| TEXAS INSTRUMENTS INCORPORATED
| Standard Linear and Logic Group
| IBIS Model of SN74CB3T16210
| 20-BIT FET BUS SWITCH 2.5-V/3.3-V LOW-VOLTAGE BUS SWITCH
| WITH 5-V TOLERANT/LEVEL SHIFTER
| This file contains package information for the following:
|  TSSOP 48-pin (DGG) package as [Component] CB3T16210_DGG
|  TVSOP 48-pin (DGV) package as [Component] CB3T16210_DGV
| This device can be powered at the following Vccs:
|  3.3 volt Vcc
|  2.5 volt Vcc
| This file provides unique models under the [Model Selector] for each Vcc.
| For operation at a specific Vcc, select the appropriate model after each
| [Model Selector] keyword.
[IBIS Ver]   3.2
[Comment char]  |_char
[File Name]   sn74cb3t16210.ibs
[File Rev]   1.1 | c_die
[Date]   April 30, 2004
[Source]   Data created from TI-SPICE simulations at TI-SLL.
[Notes]   The following is an IBIS list for the CB3T16210.
   Please contact sllibis@ti.com with questions and
   comments concerning SLL IBIS models.
   - FILE REV HISTORY
   - 1.1 Release IBIS file on 06/01/04
   - Non-monotonic data due to FET characteristics.
   - Power clamp data deleted as there is no power-clamp diode.
[Disclaimer] Property of Texas Instruments Incorporated.  Unauthorized
   reproduction and/or distribution is strictly prohibited.
   This product is protected under copyright law.
   Created  2003, (C) Copyright  2003, Texas Instruments
   Incorporated, All Rights Reserved
   UNLESS THERE IS A SIGNED, WRITTEN AGREEMENT TO THE
   CONTRARY, TEXAS INSTRUMENTS (TI) IS PROVIDING THE IBIS
   MODELS  AND WITHOUT ANY WARRANTY, EXPRESSED OR
   IMPLIED.  TI assumes no liability for:
   1) the accuracy of the IBIS models provided to your
   company;
   2) the proper functioning of these IBIS Models in your
   design or for any resulting applications; or
   3) infringement of patents, copyrights or intellectual
   property rights resulting from your use of these IBIS
   models.
   TI provides IBIS Models as a service to our customers.
   You and your company shall not distribute, sell or give
   these models to anyone else without prior written
   permission from TI.
   TI reserves the right to make changes to our products or
   to discontinue any semiconductor product or service
   without notice, and advises our customers to obtain the
   latest version of relevant information to verify, before
   placing orders, that the information being relied on is
   current.
   Please be aware that your receipt and use of the IBIS
   information provided shall serve as acceptance of these
   terms and conditions.  If you do not accept these terms,
   you should return or destroy the IBIS models and any
   other accompanying information immediately.
| Component CB3T16210_DGG 48-pin TSSOP
[Component]   CB3T16210_DGG
[Manufacturer]   Texas Instruments, Inc.
[Package]
|   typ   min   max
R_pkg   4.400e-02   3.800e-02   5.100e-02
L_pkg   3.019e-09   2.486e-09   4.099e-09
C_pkg   5.070e-13   3.340e-13   8.090e-13
[Pin]   signal_name   model_name   R_pin   L_pin   C_pin
1   NC   NC   4.100e-02   4.017e-09   7.590e-13
2   1A1   CB3T16210_IO   4.200e-02   3.737e-09   7.920e-13
3   1A2   CB3T16210_IO   4.200e-02   3.480e-09   6.610e-13
4   1A3   CB3T16210_IO   3.800e-02   3.131e-09   5.750e-13
5   1A4   CB3T16210_IO   4.700e-02   3.122e-09   5.660e-13
6   1A5   CB3T16210_IO   4.300e-02   2.948e-09   5.040e-13
7   1A6   CB3T16210_IO   4.500e-02   2.845e-09   3.970e-13
8   GND   GND   4.900e-02   2.835e-09   3.940e-13
9   1A7   CB3T16210_IO   4.800e-02   2.715e-09   3.780e-13
10   1A8   CB3T16210_IO   5.000e-02   2.664e-09   3.630e-13
11   1A9   CB3T16210_IO   5.000e-02   2.585e-09   3.480e-13
12   1A10   CB3T16210_IO   4.900e-02   2.550e-09   3.370e-13
13   2A1   CB3T16210_IO   4.900e-02   2.541e-09   3.360e-13
14   2A2   CB3T16210_IO   5.000e-02   2.574e-09   3.480e-13
15   VCC   POWER   4.900e-02   2.618e-09   3.590e-13
16   2A3   CB3T16210_IO   4.600e-02   2.671e-09   3.750e-13
17   GND   GND   4.500e-02   2.754e-09   3.890e-13
18   2A4   CB3T16210_IO   4.400e-02   2.823e-09   4.500e-13
19   2A5   CB3T16210_IO   4.200e-02   2.968e-09   5.030e-13
20   2A6   CB3T16210_IO   5.100e-02   3.108e-09   5.350e-13
21   2A7   CB3T16210_IO   4.200e-02   3.175e-09   5.870e-13
22   2A8   CB3T16210_IO   4.100e-02   3.449e-09   6.780e-13
23   2A9   CB3T16210_IO   4.400e-02   3.766e-09   8.040e-13
24   2A10   CB3T16210_IO   4.300e-02   4.065e-09   7.610e-13
25   2B10   CB3T16210_IO   4.100e-02   3.994e-09   7.570e-13
26   2B9   CB3T16210_IO   3.900e-02   3.649e-09   7.890e-13
27   2B8   CB3T16210_IO   3.800e-02   3.362e-09   6.600e-13
28   2B7   CB3T16210_IO   3.800e-02   3.082e-09   5.740e-13
29   2B6   CB3T16210_IO   4.400e-02   2.990e-09   5.220e-13
30   2B5   CB3T16210_IO   4.100e-02   2.917e-09   4.950e-13
31   2B4   CB3T16210_IO   4.300e-02   2.820e-09   4.480e-13
32   GND   GND   4.300e-02   2.699e-09   3.850e-13
33   2B3   CB3T16210_IO   4.500e-02   2.628e-09   3.720e-13
34   2B2   CB3T16210_IO   4.600e-02   2.556e-09   3.560e-13
35   2B1   CB3T16210_IO   4.600e-02   2.495e-09   3.440e-13
36   1B10   CB3T16210_IO   4.700e-02   2.487e-09   3.340e-13
37   1B9   CB3T16210_IO   4.700e-02   2.490e-09   3.350e-13
38   1B8   CB3T16210_IO   4.600e-02   2.486e-09   3.430e-13
39   1B7   CB3T16210_IO   4.500e-02   2.566e-09   3.560e-13
40   1B6   CB3T16210_IO   4.400e-02   2.639e-09   3.740e-13
41   GND   GND   4.300e-02   2.701e-09   3.860e-13
42   1B5   CB3T16210_IO   4.300e-02   2.817e-09   4.500e-13
43   1B4   CB3T16210_IO   4.100e-02   2.935e-09   5.010e-13
44   1B3   CB3T16210_IO   4.700e-02   3.035e-09   5.290e-13
45   1B2   CB3T16210_IO   4.300e-02   3.171e-09   5.890e-13
46   1B1   CB3T16210_IO   4.000e-02   3.415e-09   6.820e-13
47   NOE2   CB3T16210_IN   4.300e-02   3.741e-09   8.090e-13
48   NOE1   CB3T16210_IN   4.400e-02   4.099e-09   7.640e-13
| Component CB3T16210_DGV 48-pin TVSOP
[Component]   CB3T16210_DGV
[Manufacturer]   Texas Instruments, Inc.
[Package]
|   typ   min   max
R_pkg   7.000e-02   4.900e-02   8.500e-02
L_pkg   3.013e-09   2.743e-09   3.408e-09
C_pkg   3.710e-13   2.940e-13   5.110e-13
[Pin]   signal_name   model_name   R_pin   L_pin   C_pin
1   NC   NC   4.900e-02   3.393e-09   4.970e-13
2   1A1   CB3T16210_IO   6.000e-02   3.250e-09   5.020e-13
3   1A2   CB3T16210_IO   7.700e-02   3.310e-09   4.510e-13
4   1A3   CB3T16210_IO   8.500e-02   3.299e-09   4.040e-13
5   1A4   CB3T16210_IO   8.300e-02   3.136e-09   3.600e-13
6   1A5   CB3T16210_IO   7.700e-02   3.019e-09   3.630e-13
7   1A6   CB3T16210_IO   6.500e-02   2.882e-09   3.490e-13
8   GND   GND   6.600e-02   2.829e-09   3.140e-13
9   1A7   CB3T16210_IO   6.700e-02   2.796e-09   3.140e-13
10   1A8   CB3T16210_IO   6.900e-02   2.754e-09   3.080e-13
11   1A9   CB3T16210_IO   7.000e-02   2.753e-09   3.010e-13
12   1A10   CB3T16210_IO   7.100e-02   2.745e-09   2.940e-13
13   2A1   CB3T16210_IO   7.000e-02   2.744e-09   2.940e-13
14   2A2   CB3T16210_IO   7.000e-02   2.754e-09   3.010e-13
15   VCC   POWER   6.900e-02   2.754e-09   3.080e-13
16   2A3   CB3T16210_IO   6.700e-02   2.796e-09   3.140e-13
17   GND   GND   6.600e-02   2.829e-09   3.140e-13
18   2A4   CB3T16210_IO   6.500e-02   2.883e-09   3.500e-13
19   2A5   CB3T16210_IO   7.500e-02   3.014e-09   3.630e-13
20   2A6   CB3T16210_IO   8.000e-02   3.128e-09   3.580e-13
21   2A7   CB3T16210_IO   8.400e-02   3.295e-09   4.030e-13
22   2A8   CB3T16210_IO   7.800e-02   3.311e-09   4.520e-13
23   2A9   CB3T16210_IO   6.200e-02   3.259e-09   5.010e-13
24   2A10   CB3T16210_IO   5.200e-02   3.404e-09   4.960e-13
25   2B10   CB3T16210_IO   5.300e-02   3.397e-09   5.050e-13
26   2B9   CB3T16210_IO   6.200e-02   3.249e-09   5.110e-13
27   2B8   CB3T16210_IO   7.700e-02   3.308e-09   4.530e-13
28   2B7   CB3T16210_IO   8.200e-02   3.289e-09   4.030e-13
29   2B6   CB3T16210_IO   7.800e-02   3.121e-09   3.590e-13
30   2B5   CB3T16210_IO   7.400e-02   3.010e-09   3.630e-13
31   2B4   CB3T16210_IO   6.500e-02   2.883e-09   3.490e-13
32   GND   GND   6.700e-02   2.829e-09   3.140e-13
33   2B3   CB3T16210_IO   6.700e-02   2.795e-09   3.140e-13
34   2B2   CB3T16210_IO   6.900e-02   2.753e-09   3.070e-13
35   2B1   CB3T16210_IO   7.000e-02   2.753e-09   3.010e-13
36   1B10   CB3T16210_IO   7.000e-02   2.743e-09   2.940e-13
37   1B9   CB3T16210_IO   7.000e-02   2.743e-09   2.940e-13
38   1B8   CB3T16210_IO   7.000e-02   2.753e-09   3.010e-13
39   1B7   CB3T16210_IO   6.900e-02   2.754e-09   3.070e-13
40   1B6   CB3T16210_IO   6.800e-02   2.797e-09   3.140e-13
41   GND   GND   6.700e-02   2.830e-09   3.140e-13
42   1B5   CB3T16210_IO   6.400e-02   2.880e-09   3.490e-13
43   1B4   CB3T16210_IO   7.200e-02   3.004e-09   3.620e-13
44   1B3   CB3T16210_IO   7.800e-02   3.121e-09   3.590e-13
45   1B2   CB3T16210_IO   8.400e-02   3.296e-09   4.030e-13
46   1B1   CB3T16210_IO   7.700e-02   3.308e-09   4.510e-13
47   NOE2   CB3T16210_IN   6.200e-02   3.258e-09   4.990e-13
48   NOE1   CB3T16210_IN   5.300e-02   3.408e-09   4.940e-13
[Series Switch Groups]
| Function Group States
On  1 /   | 1A1-1A10->1B1-1B10 NOE1 LOW
On  2 /   | 2A1-2A10->2B1-2B10 NOE2 LOW
On  1 2 /   | Enable Both
Off 1 /   | 1A1-1A10->1B1-1B10 NOE1 HIGH
Off 2 /   | 2A1-2A10->2B1-2B10 NOE2 HIGH
Off 1 2 /   | Disable Both
[Series Pin Mapping]   pin_2   model_name   function_table_group
2   46   CB3T16210_IO_33_S   1
| 2   46   CB3T16210_IO_25_S   1
3   45   CB3T16210_IO_33_S   1
| 3   45   CB3T16210_IO_25_S   1
4   44   CB3T16210_IO_33_S   1
| 4   44   CB3T16210_IO_25_S   1
5   43   CB3T16210_IO_33_S   1
| 5   43   CB3T16210_IO_25_S   1
6   42   CB3T16210_IO_33_S   1
| 6   42   CB3T16210_IO_25_S   1
7   40   CB3T16210_IO_33_S   1
| 7   40   CB3T16210_IO_25_S   1
9   39   CB3T16210_IO_33_S   1
| 9   39   CB3T16210_IO_25_S   1
10   38   CB3T16210_IO_33_S   1
| 10   38   CB3T16210_IO_25_S   1
11   37   CB3T16210_IO_33_S   1
| 11   37   CB3T16210_IO_25_S   1
12   36   CB3T16210_IO_33_S   1
| 12   36   CB3T16210_IO_25_S   1
13   35   CB3T16210_IO_33_S   2
| 13   35   CB3T16210_IO_25_S   2
14   34   CB3T16210_IO_33_S   2
| 14   34   CB3T16210_IO_25_S   2
16   33   CB3T16210_IO_33_S   2
| 16   33   CB3T16210_IO_25_S   2
18   31   CB3T16210_IO_33_S   2
| 18   31   CB3T16210_IO_25_S   2
19   30   CB3T16210_IO_33_S   2
| 19   30   CB3T16210_IO_25_S   2
20   29   CB3T16210_IO_33_S   2
| 20   29   CB3T16210_IO_25_S   2
21   28   CB3T16210_IO_33_S   2
| 21   28   CB3T16210_IO_25_S   2
22   27   CB3T16210_IO_33_S   2
| 22   27   CB3T16210_IO_25_S   2
23   26   CB3T16210_IO_33_S   2
| 23   26   CB3T16210_IO_25_S   2
24   25   CB3T16210_IO_33_S   2
| 24   25   CB3T16210_IO_25_S   2
| Model CB3T16210_IN
[Model Selector]   CB3T16210_IN
CB3T16210_IN_33   3.3 volt Vcc
CB3T16210_IN_25   2.5 volt Vcc
| Model CB3T16210_IO
[Model Selector]   CB3T16210_IO
CB3T16210_IO_33   3.3 volt Vcc
CB3T16210_IO_25   2.5 volt Vcc
| Model CB3T16210_IO_S
[Model Selector]   CB3T16210_IO_S
CB3T16210_IO_33_S   3.3 volt Vcc_S
CB3T16210_IO_25_S   2.5 volt Vcc_S
[Model]   CB3T16210_IO_33_S
Model_type  Series_switch
| variable   typ   min   max
C_comp   0   0   0
[Temperature Range]   40   100   -40
| Ambient temperature   25   85   -40
[Voltage range]   3.3   3   3.6
[On]
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[Off]
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[Model]   CB3T16210_IO_25_S
Model_type  Series_switch
| variable   typ   min   max
C_comp   0   0   0
[Temperature Range]   40   100   -40
| Ambient temperature   25   85   -40
[Voltage range]   2.5   2.3   2.7
[On]
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[Off]
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| Models and submodels in the file (6): CB3T16210_IN_33 (Input), CB3T16210_IN_25 (Input), CB3T16210_IO_33_S (Series_switch), CB3T16210_IO_33 (Terminator), CB3T16210_IO_25_S (Series_switch), CB3T16210_IO_25 (Terminator)
